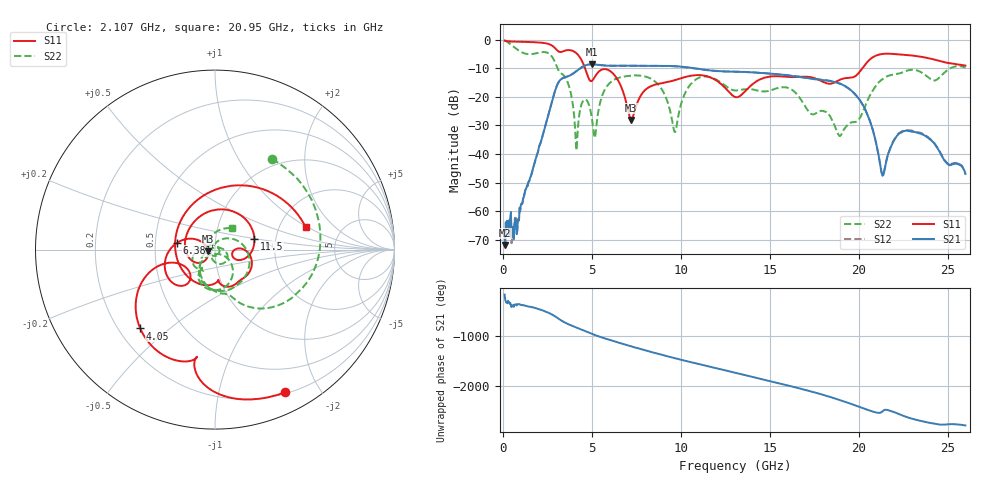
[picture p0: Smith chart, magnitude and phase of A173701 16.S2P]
!  2-Port S-parameters saved by WinCal
! VAR MeasName=S-Parameters (CALIBRATED_DATA) read from VNA (N5245A)
! VAR MeasDate=2017-6-7 10:29:24
! VAR NAME=A173701 16
! VAR FILENAME=A173701 16.S2P
! VAR DATE=2017-6-7 10:29:24
! VAR PHYS_PORTS=1,2
# Hz S DB R 50
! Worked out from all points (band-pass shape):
!   801 points, 100 MHz to 26 GHz, reference 50 ohm
!   highest |S21| = -8.63 dB at 5.021 GHz (marker M1); lowest = -71.8 dB at 132.4 MHz (marker M2)
!   |S21| within 3 dB of the highest: 4.014 GHz to 14.37 GHz (10.35 GHz wide, 113 % of centre)
!   lowest |S11| = -28.1 dB at 7.223 GHz (marker M3), VSWR 1.08, Z = 46.3 - j0.77 ohm
!   |S11| at or under -10 dB: 4.618 GHz to 20.21 GHz (15.59 GHz wide, 126 % of centre)
!   |S22| runs from -38.7 to -0.3 dB; largest |S21 - S12| = 0.005
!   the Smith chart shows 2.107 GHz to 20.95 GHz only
!   S11 on the Smith chart (normalised r, x): 2.107 GHz: 0.22, -1.58; 4.05 GHz: 0.29, -0.40; 6.381 GHz: 0.65, +0.05; 11.5 GHz: 1.55, +0.19; 20.95 GHz: 2.79, +0.97
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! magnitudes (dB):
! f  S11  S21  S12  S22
! 100 MHz  -0.3  -68.3  -72.1  -0.3
! 132.4 MHz  -0.4  -71.8  -72.2  -0.4
! 747.5 MHz  -0.8  -63.3  -62.4  -3.2
! 2.107 GHz  -1.1  -36.4  -36.3  -4.5
! 3.596 GHz  -3.7  -13.0  -12.9  -14.2
! 4.05 GHz  -4.4  -11.5  -11.4  -29.9
! 4.438 GHz  -7.4  -9.7  -9.7  -22.3
! 5.021 GHz  -14.4  -8.6  -8.6  -28.2
! 6.381 GHz  -13.3  -9.1  -9.1  -13.6
! 7.223 GHz  -28.1  -9.2  -9.1  -12.6
! 8.744 GHz  -15.5  -9.2  -9.2  -15.8
! 9.683 GHz  -14.2  -9.3  -9.4  -32.3
! 10.4 GHz  -12.9  -9.7  -9.8  -17.0
! 11.5 GHz  -12.9  -10.7  -10.7  -12.9
! 13.05 GHz  -20.0  -11.2  -11.2  -17.8
! 17.39 GHz  -13.2  -13.8  -13.6  -26.1
! 18.97 GHz  -14.0  -15.5  -15.4  -33.6
! 20.95 GHz  -5.7  -35.3  -35.3  -16.4
! 21.34 GHz  -5.0  -47.6  -47.3  -13.8
! 21.69 GHz  -4.9  -39.4  -39.3  -12.6
! 23.41 GHz  -5.9  -32.7  -32.5  -11.1
! 26 GHz  -9.1  -46.9  -47.1  -9.9
